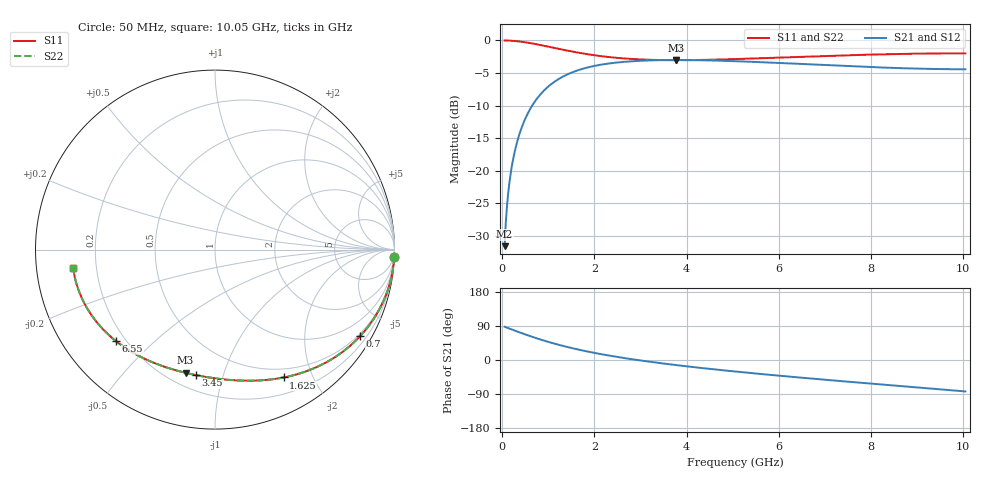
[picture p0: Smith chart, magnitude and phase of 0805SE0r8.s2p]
! AVX Thin Film Operation		Date: August 2001
! Description: Accu-P® Series, Thin Film, SMD, RF Capacitor
! Part Number: 08051J0R8ABT
! 50 MHz  -  10.05 GHz
! Serial Measurements
# mhz S db R 50
!	S11		S21		S12		S22
!	dB	Phase	dB	Phase	dB	Phase	dB	Phase
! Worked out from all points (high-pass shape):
!   401 points, 50 MHz to 10.05 GHz, reference 50 ohm
!   highest |S21| = -3.00 dB at 3.775 GHz (marker M1); lowest = -31.5 dB at 50 MHz (marker M2)
!   |S21| within 3 dB of the highest: 1.203 GHz to end of sweep
!   lowest |S11| = -3.0 dB at 3.775 GHz (marker M3), VSWR 5.80, Z = 13.7 - j37.6 ohm
!   |S11| at or under -10 dB: nowhere
!   |S22| runs from -3.0 to 0.0 dB; largest |S21 - S12| = 7.8e-05
!   S11 on the Smith chart (normalised r, x): 50 MHz: 0, -50; 700 MHz: 0.42, -3.57; 1.625 GHz: 0.39, -1.60; 3.45 GHz: 0.29, -0.82; 6.55 GHz: 0.16, -0.38; 10.05 GHz: 0.11, -0.06
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50  -0.00 -2.3  -31.55 87.7  -31.55 87.7  -0.00 -2.3
150  -0.03 -6.9  -22.04 83.1  -22.04 83.1  -0.03 -6.9
200  -0.05 -9.2  -19.57 80.8  -19.57 80.8  -0.05 -9.2
275  -0.09 -12.6  -16.87 77.4  -16.87 77.4  -0.09 -12.6
350  -0.14 -16.0  -14.86 74.0  -14.86 74.0  -0.14 -16.0
450  -0.23 -20.4  -12.81 69.6  -12.81 69.6  -0.23 -20.4
700  -0.53 -30.9  -9.43 59.1  -9.43 59.1  -0.53 -30.9
900  -0.81 -38.6  -7.71 51.4  -7.71 51.4  -0.81 -38.6
1125  -1.14 -46.6  -6.37 43.4  -6.37 43.4  -1.14 -46.6
1625  -1.84 -61.8  -4.61 28.2  -4.61 28.2  -1.84 -61.8
1725  -1.97 -64.5  -4.39 25.5  -4.39 25.5  -1.97 -64.4
2075  -2.35 -73.0  -3.80 17.0  -3.80 17.0  -2.35 -73.0
2475  -2.66 -81.5  -3.40 8.5  -3.40 8.5  -2.66 -81.5
2900  -2.88 -89.5  -3.15 0.5  -3.15 0.5  -2.88 -89.5
3400  -3.00 -97.8  -3.03 -7.8  -3.03 -7.8  -3.00 -97.8
3450  -3.01 -98.5  -3.02 -8.6  -3.02 -8.6  -3.01 -98.5
3775  -3.03 -103.4  -3.00 -13.5  -3.00 -13.5  -3.03 -103.4
5050  -2.86 -120.2  -3.18 -30.3  -3.18 -30.3  -2.86 -120.2
6550  -2.49 -137.2  -3.62 -47.3  -3.62 -47.3  -2.49 -137.2
6725  -2.44 -139.1  -3.68 -49.2  -3.68 -49.2  -2.44 -139.1
8400  -2.10 -156.2  -4.19 -66.3  -4.19 -66.3  -2.10 -156.2
10050  -1.97 -172.8  -4.42 -83.0  -4.42 -83.0  -1.97 -172.8
